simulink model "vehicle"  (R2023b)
settings: Solver=ode3  StartTime=0.0  StopTime=t_end  FixedStep=dt8dof  RelTol=1e-3
PreLoadFcn:
  | define_swarm_buses(3, 1000);
model workspace (MAT data in the model file):
  Af = 1.8
  Cp_tyre = 500
  Cx = 0.28
  G = 15000
  Ha = 0.4
  Hg = 0.4
  Hroll = 0.304
  Hroll_f = 0.08
  Hroll_r = 0.12
  Ir = 0.8
  Ix = 450
  Jz = 1800
  K = 130000
  K_psi = 0.48
  K_y = 0.06
  Karb_F = 26000
  Karb_R = 26000
  KdF = 0
  KdR = 0
  Kd_h = 0
  Kd_v = 0
  Kd_y = 0
  Ki_h = 0
  Ki_v = 0.1
  Ki_y = 0
  Kp_h = 1.5
  Kp_v = 1.5
  Kp_y = 0.1
  Ks_f = 39000
  Ks_r = 39000
  Kv = 290000
  L = 1.5
  Lril_L = 0.055
  Lril_T = 0.5
  MAX_PATH_LEN = 1000
  Pacn = [3000 1 1 1 1 1 1 1 1 0 0 0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]
  R0 = 0.2
  Rfront = 0.2
  Rr_sterzo = 0
  Rrear = 0.2
  Rs = 13
  Tf = 1.5
  Tr = 1.5
  a = 0.6
  a_brake = -3
  b = 0.9
  camb_0F = 0
  camb_0R = -0.00680678408278
  d_max = 0.558505360638
  dt8dof = 0.002
  dtastar = 0.1
  dtcontrol = 0.03
  f0 = 0.0041
  f2 = 2.051e-07
  g = 9.81
  m = 1300
  mot_T_table = [0 0 0 0 0 0 0 0 0 0 0 0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]
  mot_alpha_bp = [0 10 20 30 40 50 60 70 80 90 100]
  mot_n_bp = [0 29.9163426864 59.8326853729 89.7490280593 119.665370746 149.581713432 179.498056119 209.414398805 239.330741492 269.247084178 299.163426864 329.079769551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]
  mpc_speed : object (value not decoded)
  phi_road0 = 0
  psi0 = 0
  r_goal = 5
  r_slow = 30
  replan_steps = 20
  rho = 1.3
  slope_x_body0 = 0
  slope_y_body0 = 0
  t_end = 70
  terrain_truth_mu_table = [-1 -1 -1 -1 -1 -1 -1 -1 -1 -1 -1 -1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]
  terrain_truth_obstacle_table = [1 1 1 1 1 1 1 1 1 1 1 1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]
  terrain_truth_slope_deg_table = [2.67415653197 2.67413215857 2.67406695826 2.6739952249 2.6739164067 2.67382991742 2.67373513563 2.67363140411 2.67351802953 2.67339428225 2.67325939642 2.67311257041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]
  terrain_truth_slope_x_table = [-0.0458815772305 -0.0458808922252 -0.0458794511544 -0.0458778616187 -0.0458761104845 -0.0458741837099 -0.0458720663111 -0.0458697423295 -0.0458671948025 -0.0458644057365 -0.0458613560839 -0.045858025724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]
  terrain_truth_slope_y_table = [0.00874081815183 0.00874213563744 0.00874360556 0.00874524373283 0.00874706738108 0.00874909524079 0.00875134766185 0.00875384671474 0.00875661630067 0.00875968226488 0.00876307251276 0.0087668171283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]
  terrain_truth_traversable_table = [0 0 0 0 0 0 0 0 0 0 0 0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]
  terrain_truth_x_bp = [0 1 2 3 4 5 6 7 8 9 10 11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]
  terrain_truth_y_bp = [0 1 2 3 4 5 6 7 8 9 10 11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]
  teta0 = 0
  tetapunto0 = 0
  theta_road0 = 0
  toe_F = -0.00174532925199
  toe_R = 0.00174532925199
  velstart = 5
  wr0_FL = 3.15
  wr0_FR = 3.15
  wr0_RL = 3.15
  wr0_RR = 3.15
  x0 = 0
  y0 = 0
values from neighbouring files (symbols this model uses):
  gear_ratio = 10    [motor_map.m]
  v_ref_init = scenario.vehicle8.velstart    [make_vref_filter.m]
undefined symbols (not defined in the file or in its folder): A_f, B_f, C_f, D_f, psi0_1
libraries: simulink_extras x15, mpclib x1, slpidlib x1
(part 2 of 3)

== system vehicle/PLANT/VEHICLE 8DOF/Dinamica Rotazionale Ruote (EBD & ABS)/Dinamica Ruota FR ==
  Cm : Inport
  Cf : Inport  Port=2
  Fx : Inport  Port=3
  R : Inport  Port=4
  Fz : Inport  Port=5
  Rr : Inport  Port=6
  Add : Sum  Inputs=+---
  Constant : Constant  Value=velstart
  Divide : Product  Inputs=*/
  FR : Scope
  Integrator2 : Integrator  InitialConditionSource=external  LowerSaturationLimit=0
  Manual Switch : ManualSwitch  CurrentSetting=0
  Mom Inerzia Ruota : Constant  Value=Ir
  Mux : Mux  Inputs=5
  Mux2 : Mux  Inputs=2
  Product3 : Product  RndMeth=Zero
  Product5 : Product  Inputs=*/  RndMeth=Zero
  Resistenza a Rotolmento : Fcn  Expr=u(1)*(f0+f2*u(2)^2)
  Saturation : Saturate  UpperLimit=inf  LowerLimit=0
  cond iniziale wr0 : Constant  Value=wr0_FR
  w : Outport  VectorParamsAs1DForOutWhenUnconnected=off
  R_roll : Outport  Port=2
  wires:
  Resistenza a Rotolmento/1 -> R_roll/1, Add/4, Mux/5
  Mux2/1 -> Resistenza a Rotolmento/1
  Integrator2/1 -> Mux2/2, Saturation/1
  Fz/1 -> Mux2/1
  Product5/1 -> Integrator2/1
  Mom Inerzia Ruota/1 -> Product5/2
  Add/1 -> Product5/1
  Product3/1 -> Add/3, Mux/3
  R/1 -> Product3/2, Mux/4
  Fx/1 -> Product3/1
  Cf/1 -> Add/2, Mux/2
  Cm/1 -> Add/1, Mux/1
  Mux/1 -> FR/1
  Manual Switch/1 -> Integrator2/2
  cond iniziale wr0/1 -> Manual Switch/1
  Saturation/1 -> w/1
  Divide/1 -> Manual Switch/2
  Rr/1 -> Divide/2
  Constant/1 -> Divide/1

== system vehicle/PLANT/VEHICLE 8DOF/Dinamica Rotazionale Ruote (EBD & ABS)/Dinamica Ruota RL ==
  Cm : Inport
  Cf : Inport  Port=2
  Fx : Inport  Port=3
  R : Inport  Port=4
  Fz : Inport  Port=5
  Rr : Inport  Port=6
  Add : Sum  Inputs=+---
  Constant : Constant  Value=velstart
  Divide : Product  Inputs=*/
  Integrator2 : Integrator  InitialConditionSource=external  LowerSaturationLimit=0
  Manual Switch : ManualSwitch  CurrentSetting=0
  Mom Inerzia Ruota : Constant  Value=Ir
  Mux : Mux  Inputs=5
  Mux2 : Mux  Inputs=2
  Product3 : Product  RndMeth=Zero
  Product5 : Product  Inputs=*/  RndMeth=Zero
  RL : Scope
  Resistenza a Rotolmento : Fcn  Expr=u(1)*(f0+f2*u(2)^2)
  Saturation : Saturate  UpperLimit=inf  LowerLimit=0
  cond iniziale wr0 : Constant  Value=wr0_RL
  w : Outport  VectorParamsAs1DForOutWhenUnconnected=off
  R_roll : Outport  Port=2
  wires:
  Resistenza a Rotolmento/1 -> R_roll/1, Add/4, Mux/5
  Mux2/1 -> Resistenza a Rotolmento/1
  Integrator2/1 -> Mux2/2, Saturation/1
  Fz/1 -> Mux2/1
  Product5/1 -> Integrator2/1
  Mom Inerzia Ruota/1 -> Product5/2
  Add/1 -> Product5/1
  Product3/1 -> Add/3
  R/1 -> Product3/2, Mux/4
  Fx/1 -> Mux/3, Product3/1
  Cf/1 -> Add/2, Mux/2
  Cm/1 -> Add/1, Mux/1
  Mux/1 -> RL/1
  Manual Switch/1 -> Integrator2/2
  cond iniziale wr0/1 -> Manual Switch/1
  Saturation/1 -> w/1
  Divide/1 -> Manual Switch/2
  Rr/1 -> Divide/2
  Constant/1 -> Divide/1

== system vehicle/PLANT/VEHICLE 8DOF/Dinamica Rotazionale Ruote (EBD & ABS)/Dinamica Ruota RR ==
  Cm : Inport
  Cf : Inport  Port=2
  Fx : Inport  Port=3
  R : Inport  Port=4
  Fz : Inport  Port=5
  Rr : Inport  Port=6
  Add : Sum  Inputs=+---
  Constant : Constant  Value=velstart
  Divide : Product  Inputs=*/
  Integrator2 : Integrator  InitialConditionSource=external  LowerSaturationLimit=0
  Manual Switch : ManualSwitch  CurrentSetting=0
  Mom Inerzia Ruota : Constant  Value=Ir
  Mux : Mux  Inputs=5
  Mux2 : Mux  Inputs=2
  Product3 : Product  RndMeth=Zero
  Product5 : Product  Inputs=*/  RndMeth=Zero
  RR : Scope
  Resistenza a Rotolmento : Fcn  Expr=u(1)*(f0+f2*u(2)^2)
  Saturation : Saturate  UpperLimit=inf  LowerLimit=0
  cond iniziale wr0 : Constant  Value=wr0_RR
  w : Outport  VectorParamsAs1DForOutWhenUnconnected=off
  R_roll : Outport  Port=2
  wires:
  Resistenza a Rotolmento/1 -> R_roll/1, Add/4, Mux/5
  Mux2/1 -> Resistenza a Rotolmento/1
  Integrator2/1 -> Mux2/2, Saturation/1
  Fz/1 -> Mux2/1
  Product5/1 -> Integrator2/1
  Mom Inerzia Ruota/1 -> Product5/2
  Add/1 -> Product5/1
  Product3/1 -> Add/3
  R/1 -> Product3/2, Mux/4
  Fx/1 -> Mux/3, Product3/1
  Cf/1 -> Add/2, Mux/2
  Cm/1 -> Add/1, Mux/1
  Mux/1 -> RR/1
  Manual Switch/1 -> Integrator2/2
  cond iniziale wr0/1 -> Manual Switch/1
  Saturation/1 -> w/1
  Divide/1 -> Manual Switch/2
  Rr/1 -> Divide/2
  Constant/1 -> Divide/1

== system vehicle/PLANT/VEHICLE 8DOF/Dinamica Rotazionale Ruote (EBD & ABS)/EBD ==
  %brake : Inport
  mu : Inport  Port=2
  Fz : Inport  Port=3
  Add : Sum  Inputs=++++
  Demux : Demux
  Divide{,1..3} (4 alike) : Product  Inputs=*/
  Gain : Gain  Gain=1.5
  Mux : Mux
  Product{,1..4} (5 alike) : Product
  Saturation : Saturate  UpperLimit=inf  LowerLimit=.05
  Saturation1 : Saturate  UpperLimit=inf  LowerLimit=50
  Saturation2 : Saturate  UpperLimit=inf  LowerLimit=eps
  Cf : Outport
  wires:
  mu/1 -> Saturation/1
  Fz/1 -> Saturation1/1
  Product/1 -> Demux/1
  Demux/1 -> Divide/1, Add/1
  Saturation/1 -> Product/1
  Saturation1/1 -> Product/2
  Demux/2 -> Divide1/1, Add/2
  Demux/3 -> Divide2/1, Add/3
  Demux/4 -> Divide3/1, Add/4
  Add/1 -> Saturation2/1
  Saturation2/1 -> Divide3/2, Divide2/2, Divide1/2, Divide/2
  Divide/1 -> Product1/1
  %brake/1 -> Product4/2, Product3/2, Product2/2, Product1/2
  Divide1/1 -> Product2/1
  Divide2/1 -> Product3/1
  Divide3/1 -> Product4/1
  Product1/1 -> Mux/1
  Product2/1 -> Mux/2
  Product3/1 -> Mux/3
  Product4/1 -> Mux/4
  Mux/1 -> Gain/1
  Gain/1 -> Cf/1

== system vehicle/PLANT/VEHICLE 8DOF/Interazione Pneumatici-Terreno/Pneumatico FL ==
  vel_x : Inport
  R : Inport  Port=2
  alfa : Inport  Port=3
  Fz : Inport  Port=4
  mu_strada : Inport  Port=5
  w : Inport  Port=6
  Calcolo FORZA LATERALE & LONGITUDINALE (Pneumatico - Terreno) : Subsystem
  Gain : Gain  Gain=-1
  Lunghezze di rilassamento : Subsystem
  Radians to Degrees : simulink_extras/Transformations/Radians to Degrees
  Scorrimento : Subsystem
  Fx_rit : Outport  VectorParamsAs1DForOutWhenUnconnected=off
  Fy_rit : Outport  Port=2  VectorParamsAs1DForOutWhenUnconnected=off
  slip_FL : Outport  Port=3
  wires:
  vel_x/1 -> Scorrimento/1(vel_x_cr), Lunghezze di rilassamento/1(vel_x_CR), Calcolo FORZA LATERALE & LONGITUDINALE (Pneumatico - Terreno)/1(Vcx)
  R/1 -> Scorrimento/2(R)
  w/1 -> Scorrimento/3(w)
  Calcolo FORZA LATERALE & LONGITUDINALE (Pneumatico - Terreno)/1(Fy) -> Lunghezze di rilassamento/2(Fy)
  Calcolo FORZA LATERALE & LONGITUDINALE (Pneumatico - Terreno)/2(Fx) -> Lunghezze di rilassamento/3(Fx)
  Scorrimento/1(s) -> slip_FL/1, Calcolo FORZA LATERALE & LONGITUDINALE (Pneumatico - Terreno)/3(s)
  alfa/1 -> Radians to Degrees/1
  Fz/1 -> Calcolo FORZA LATERALE & LONGITUDINALE (Pneumatico - Terreno)/4(Fz)
  Lunghezze di rilassamento/1(Fy_rit) -> Gain/1
  mu_strada/1 -> Calcolo FORZA LATERALE & LONGITUDINALE (Pneumatico - Terreno)/2(mu_strada)
  Radians to Degrees/1 -> Calcolo FORZA LATERALE & LONGITUDINALE (Pneumatico - Terreno)/5(alfa)
  Gain/1 -> Fy_rit/1
  Lunghezze di rilassamento/2(Fx_rit) -> Fx_rit/1

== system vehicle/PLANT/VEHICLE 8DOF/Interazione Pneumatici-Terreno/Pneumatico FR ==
  vel_x : Inport
  R : Inport  Port=2
  alfa : Inport  Port=3
  Fz : Inport  Port=4
  mu_strada : Inport  Port=5
  w : Inport  Port=6
  Calcolo FORZA LATERALE & LONGITUDINALE (Pneumatico - Terreno) : Subsystem
  First Order Hold1 : FirstOrderHold  Commented=through  ErrorTolerance=inf  AllowContinuousInput=on
  First Order Hold2 : FirstOrderHold  Commented=through  ErrorTolerance=inf  AllowContinuousInput=on
  Gain : Gain  Gain=-1
  Lunghezze di rilassamento : Subsystem
  Radians to Degrees : simulink_extras/Transformations/Radians to Degrees
  Scorrimento : Subsystem
  Fx_rit : Outport  VectorParamsAs1DForOutWhenUnconnected=off
  Fy_rit : Outport  Port=2  VectorParamsAs1DForOutWhenUnconnected=off
  slip_FR : Outport  Port=3
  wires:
  vel_x/1 -> Scorrimento/1(vel_x_cr), Calcolo FORZA LATERALE & LONGITUDINALE (Pneumatico - Terreno)/1(Vcx), Lunghezze di rilassamento/1(vel_x_CR)
  R/1 -> Scorrimento/2(R)
  w/1 -> Scorrimento/3(w)
  Calcolo FORZA LATERALE & LONGITUDINALE (Pneumatico - Terreno)/1(Fy) -> Lunghezze di rilassamento/2(Fy)
  Calcolo FORZA LATERALE & LONGITUDINALE (Pneumatico - Terreno)/2(Fx) -> Lunghezze di rilassamento/3(Fx)
  Scorrimento/1(s) -> slip_FR/1, Calcolo FORZA LATERALE & LONGITUDINALE (Pneumatico - Terreno)/3(s)
  alfa/1 -> Radians to Degrees/1
  Fz/1 -> Calcolo FORZA LATERALE & LONGITUDINALE (Pneumatico - Terreno)/4(Fz)
  Lunghezze di rilassamento/1(Fy_rit) -> Gain/1
  Lunghezze di rilassamento/2(Fx_rit) -> First Order Hold2/1
  mu_strada/1 -> Calcolo FORZA LATERALE & LONGITUDINALE (Pneumatico - Terreno)/2(mu_strada)
  Radians to Degrees/1 -> Calcolo FORZA LATERALE & LONGITUDINALE (Pneumatico - Terreno)/5(alfa)
  Gain/1 -> First Order Hold1/1
  First Order Hold1/1 -> Fy_rit/1
  First Order Hold2/1 -> Fx_rit/1

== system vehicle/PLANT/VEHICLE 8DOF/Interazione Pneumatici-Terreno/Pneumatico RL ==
  vel_x : Inport
  R : Inport  Port=2
  alfa : Inport  Port=3
  Fz : Inport  Port=4
  mu_strada : Inport  Port=5
  w : Inport  Port=6
  Calcolo FORZA LATERALE & LONGITUDINALE (Pneumatico - Terreno) : Subsystem
  First Order Hold1 : FirstOrderHold  Commented=through  ErrorTolerance=inf  AllowContinuousInput=on
  First Order Hold2 : FirstOrderHold  Commented=through  ErrorTolerance=inf  AllowContinuousInput=on
  Gain : Gain  Gain=-1
  Lunghezze di rilassamento : Subsystem
  Radians to Degrees : simulink_extras/Transformations/Radians to Degrees
  Scorrimento : Subsystem
  Fx_rit : Outport  VectorParamsAs1DForOutWhenUnconnected=off
  Fy_rit : Outport  Port=2  VectorParamsAs1DForOutWhenUnconnected=off
  slip_RL : Outport  Port=3
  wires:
  vel_x/1 -> Scorrimento/1(vel_x_cr), Calcolo FORZA LATERALE & LONGITUDINALE (Pneumatico - Terreno)/1(Vcx), Lunghezze di rilassamento/1(vel_x_CR)
  R/1 -> Scorrimento/2(R)
  w/1 -> Scorrimento/3(w)
  Calcolo FORZA LATERALE & LONGITUDINALE (Pneumatico - Terreno)/1(Fy) -> Lunghezze di rilassamento/2(Fy)
  Calcolo FORZA LATERALE & LONGITUDINALE (Pneumatico - Terreno)/2(Fx) -> Lunghezze di rilassamento/3(Fx)
  Scorrimento/1(s) -> slip_RL/1, Calcolo FORZA LATERALE & LONGITUDINALE (Pneumatico - Terreno)/3(s)
  alfa/1 -> Radians to Degrees/1
  Fz/1 -> Calcolo FORZA LATERALE & LONGITUDINALE (Pneumatico - Terreno)/4(Fz)
  Lunghezze di rilassamento/1(Fy_rit) -> Gain/1
  Lunghezze di rilassamento/2(Fx_rit) -> First Order Hold2/1
  mu_strada/1 -> Calcolo FORZA LATERALE & LONGITUDINALE (Pneumatico - Terreno)/2(mu_strada)
  Radians to Degrees/1 -> Calcolo FORZA LATERALE & LONGITUDINALE (Pneumatico - Terreno)/5(alfa)
  Gain/1 -> First Order Hold1/1
  First Order Hold1/1 -> Fy_rit/1
  First Order Hold2/1 -> Fx_rit/1

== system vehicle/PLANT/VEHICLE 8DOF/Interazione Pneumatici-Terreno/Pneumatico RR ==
  vel_x : Inport
  R : Inport  Port=2
  alfa : Inport  Port=3
  Fz : Inport  Port=4
  mu_strada : Inport  Port=5
  w : Inport  Port=6
  Calcolo FORZA LATERALE & LONGITUDINALE (Pneumatico - Terreno) : Subsystem
  First Order Hold1 : FirstOrderHold  Commented=through  ErrorTolerance=inf  AllowContinuousInput=on
  First Order Hold2 : FirstOrderHold  Commented=through  ErrorTolerance=inf  AllowContinuousInput=on
  Gain : Gain  Gain=-1
  Lunghezze di rilassamento : Subsystem
  Radians to Degrees : simulink_extras/Transformations/Radians to Degrees
  Scorrimento : Subsystem
  Fx_rit : Outport  VectorParamsAs1DForOutWhenUnconnected=off
  Fy_rit : Outport  Port=2  VectorParamsAs1DForOutWhenUnconnected=off
  slip_RR : Outport  Port=3
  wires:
  vel_x/1 -> Scorrimento/1(vel_x_cr), Calcolo FORZA LATERALE & LONGITUDINALE (Pneumatico - Terreno)/1(Vcx), Lunghezze di rilassamento/1(vel_x_CR)
  R/1 -> Scorrimento/2(R)
  w/1 -> Scorrimento/3(w)
  Calcolo FORZA LATERALE & LONGITUDINALE (Pneumatico - Terreno)/1(Fy) -> Lunghezze di rilassamento/2(Fy)
  Calcolo FORZA LATERALE & LONGITUDINALE (Pneumatico - Terreno)/2(Fx) -> Lunghezze di rilassamento/3(Fx)
  Scorrimento/1(s) -> slip_RR/1, Calcolo FORZA LATERALE & LONGITUDINALE (Pneumatico - Terreno)/3(s)
  alfa/1 -> Radians to Degrees/1
  Fz/1 -> Calcolo FORZA LATERALE & LONGITUDINALE (Pneumatico - Terreno)/4(Fz)
  Lunghezze di rilassamento/1(Fy_rit) -> Gain/1
  Lunghezze di rilassamento/2(Fx_rit) -> First Order Hold2/1
  mu_strada/1 -> Calcolo FORZA LATERALE & LONGITUDINALE (Pneumatico - Terreno)/2(mu_strada)
  Radians to Degrees/1 -> Calcolo FORZA LATERALE & LONGITUDINALE (Pneumatico - Terreno)/5(alfa)
  Gain/1 -> First Order Hold1/1
  First Order Hold1/1 -> Fy_rit/1
  First Order Hold2/1 -> Fx_rit/1

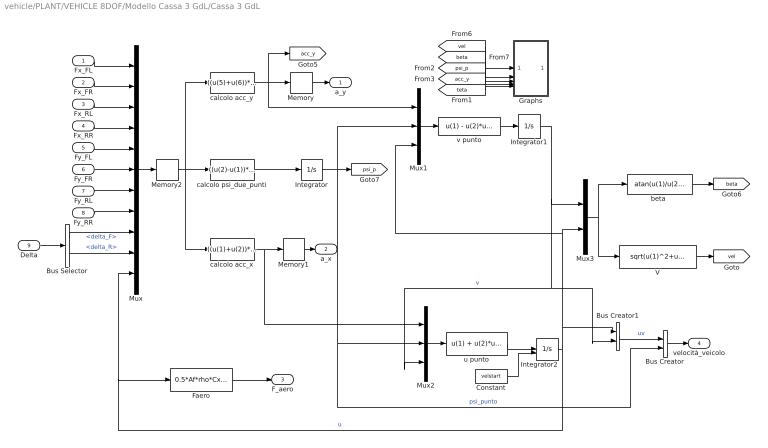
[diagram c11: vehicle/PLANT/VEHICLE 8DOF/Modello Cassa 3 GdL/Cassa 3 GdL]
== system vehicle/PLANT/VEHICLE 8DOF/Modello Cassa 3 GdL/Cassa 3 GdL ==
  Fx_FL : Inport
  Fx_FR : Inport  Port=2
  Fx_RL : Inport  Port=3
  Fx_RR : Inport  Port=4
  Fy_FL : Inport  Port=5
  Fy_FR : Inport  Port=6
  Fy_RL : Inport  Port=7
  Fy_RR : Inport  Port=8
  Delta : Inport  Port=9
  Bus Creator : BusCreator  Inputs=2
  Bus Creator1 : BusCreator  Inputs=2
  Bus Selector : BusSelector  OutputSignals=delta_F,delta_R
  Constant : Constant  Value=velstart
  Faero : Fcn  Expr=0.5*Af*rho*Cx*u^2
  Graphs : Subsystem  Commented=on
  Integrator : Integrator
  Integrator1 : Integrator
  Integrator2 : Integrator  InitialConditionSource=external  InitialCondition=velstart  LimitOutput=on  LowerSaturationLimit=eps
  Memory : Memory  Commented=through
  Memory1 : Memory  Commented=through
  Memory2 : Memory  Commented=through
  Mux : Mux  Inputs=11
  Mux1 : Mux  Inputs=3
  Mux2 : Mux  Inputs=3
  Mux3 : Mux  Inputs=2
  V : Fcn  Expr=sqrt(u(1)^2+u(2)^2)
  "beta " : Fcn  Expr=atan(u(1)/u(2))
  calcolo acc_x : Fcn  Expr=((u(1)+u(2))*cos(u(9))+(u(3)+u(4))*cos(u(10))-(u(5)+u(6))*sin(u(9))-(u(7)+u(8))*sin(u(10))-(0.5*Af*rho*Cx*(u(11)^2)))/m
  calcolo acc_y : Fcn  Expr=((u(5)+u(6))*cos(u(9))+(u(7)+u(8))*cos(u(10))+(u(1)+u(2))*sin(u(9))+(u(3)+u(4))*sin(u(10)))/m
  calcolo psi_due_punti : Fcn  Expr=((u(2)-u(1))*(Tf/2)*cos(u(9))+(u(4)-u(3))*(Tr/2)*cos(u(10))+(u(1)+u(2))*a*sin(u(9))-(u(3)+u(4))*b*sin(u(10))+(u(6)+u(5))*a*cos(u(9))-(u(7)+u(8))*b*cos(u(10))-(u(6)-u(5))*(Tf/2)*sin(u(9))+(u(7)-u(8))*(Tr/2)*sin(u(10)))/Jz
  u punto : Fcn  Expr=u(1) + u(2)*u(3)
  v punto : Fcn  Expr=u(1) - u(2)*u(3)
  a_y : Outport  VectorParamsAs1DForOutWhenUnconnected=off
  a_x : Outport  Port=2  VectorParamsAs1DForOutWhenUnconnected=off
  F_aero : Outport  Port=3  VectorParamsAs1DForOutWhenUnconnected=off
  velocità_veicolo : Outport  Port=4
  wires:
  Fx_FL/1 -> Mux/1
  Fx_FR/1 -> Mux/2
  Fx_RL/1 -> Mux/3
  Fx_RR/1 -> Mux/4
  Fy_FL/1 -> Mux/5
  Fy_FR/1 -> Mux/6
  Fy_RL/1 -> Mux/7
  Fy_RR/1 -> Mux/8
  Bus Selector/2 -> Mux/10  "<delta_R>"
  Mux/1 -> Memory2/1
  calcolo acc_y/1 -> [acc_y], Mux1/1, Memory/1
  calcolo psi_due_punti/1 -> Integrator/1
  calcolo acc_x/1 -> Mux2/1, Memory1/1
  Mux2/1 -> u punto/1
  Mux1/1 -> v punto/1
  u punto/1 -> Integrator2/1
  v punto/1 -> Integrator1/1
  Mux3/1 -> "beta "/1, V/1
  V/1 -> [vel]
  Memory/1 -> a_y/1
  Memory1/1 -> a_x/1
  Faero/1 -> F_aero/1
  Bus Creator/1 -> velocità_veicolo/1
  Bus Creator1/1 -> Bus Creator/1  "uv"
  Integrator1/1 -> Mux3/1, Bus Creator1/2, Mux2/3  "v"
  Integrator2/1 -> Bus Creator1/1, Mux1/3, Mux3/2, Mux/11, Faero/1  "u"
  Integrator/1 -> [psi_p], Mux2/2, Bus Creator/2, Mux1/2  "psi_punto"
  [psi_p] -> Graphs/3(psi_p)
  [vel] -> Graphs/1(vel)
  [beta] -> Graphs/2(beta)
  [teta] -> Graphs/5(teta)
  [acc_y] -> Graphs/4(a_y)
  "beta "/1 -> [beta]
  Delta/1 -> Bus Selector/1
  Bus Selector/1 -> Mux/9  "<delta_F>"
  Constant/1 -> Integrator2/2
  Memory2/1 -> calcolo psi_due_punti/1, calcolo acc_y/1, calcolo acc_x/1

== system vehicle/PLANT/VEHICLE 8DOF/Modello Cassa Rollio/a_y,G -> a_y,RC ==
  teta_pp : Inport
  a_y,G : Inport  Port=2
  "teta " : Inport  Port=3
  Add2 : Sum
  "Distanza CG-CR " : Constant  Value=Hroll
  Divide : Product  Inputs=***
  Trigonometric Function2 : Trigonometry  Operator=cos
  a_y,RC : Outport  VectorParamsAs1DForOutWhenUnconnected=off
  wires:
  Trigonometric Function2/1 -> Divide/3
  "Distanza CG-CR "/1 -> Divide/2
  teta_pp/1 -> Divide/1
  "teta "/1 -> Trigonometric Function2/1
  a_y,G/1 -> Add2/1
  Divide/1 -> Add2/2
  Add2/1 -> a_y,RC/1

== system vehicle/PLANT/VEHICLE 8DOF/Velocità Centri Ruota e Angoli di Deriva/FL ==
  delta : Inport
  u_cr : Inport  Port=2
  v_cr : Inport  Port=3
  Add : Sum  Inputs=-+
  Mux2 : Mux  Inputs=2
  Product : Product  RndMeth=Zero
  Scope{,1..4} (5 alike) : Scope
  Trigonometric Function : Trigonometry  Operator=cos
  "V_cr " : Fcn  Expr=sqrt(u(1)^2+u(2)^2)
  num atan1 : Fcn  Expr=atan (u(2)/u(1))
  alfa : Outport  VectorParamsAs1DForOutWhenUnconnected=off
  vel_x_cr : Outport  Port=2  VectorParamsAs1DForOutWhenUnconnected=off
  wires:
  v_cr/1 -> Scope3/1, Mux2/2
  u_cr/1 -> Scope2/1, Mux2/1
  Mux2/1 -> num atan1/1, "V_cr "/1
  num atan1/1 -> Scope4/1, Add/2  "gamma"
  Add/1 -> alfa/1, Trigonometric Function/1, Scope1/1
  Trigonometric Function/1 -> Product/1
  "V_cr "/1 -> Product/2  "V_cr"
  Product/1 -> vel_x_cr/1
  delta/1 -> Scope/1, Add/1

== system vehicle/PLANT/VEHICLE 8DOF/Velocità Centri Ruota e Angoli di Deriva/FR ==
  delta : Inport
  u_cr : Inport  Port=2
  v_cr : Inport  Port=3
  Add : Sum  Inputs=-+
  Mux2 : Mux  Inputs=2
  Product : Product  RndMeth=Zero
  Trigonometric Function : Trigonometry  Operator=cos
  "V_cr " : Fcn  Expr=sqrt(u(1)^2+u(2)^2)
  num atan1 : Fcn  Expr=atan (u(2)/u(1))
  alfa : Outport  VectorParamsAs1DForOutWhenUnconnected=off
  vel_x_cr : Outport  Port=2  VectorParamsAs1DForOutWhenUnconnected=off
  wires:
  v_cr/1 -> Mux2/2
  u_cr/1 -> Mux2/1
  delta/1 -> Add/1
  Mux2/1 -> num atan1/1, "V_cr "/1
  num atan1/1 -> Add/2  "gamma"
  Add/1 -> Trigonometric Function/1, alfa/1
  Trigonometric Function/1 -> Product/1
  "V_cr "/1 -> Product/2  "V_cr"
  Product/1 -> vel_x_cr/1

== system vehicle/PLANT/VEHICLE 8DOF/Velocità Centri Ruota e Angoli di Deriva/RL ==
  delta : Inport
  u_cr : Inport  Port=2
  v_cr : Inport  Port=3
  Add : Sum  Inputs=-+
  Mux2 : Mux  Inputs=2
  Product : Product  RndMeth=Zero
  Trigonometric Function : Trigonometry  Operator=cos
  "V_cr " : Fcn  Expr=sqrt(u(1)^2+u(2)^2)
  num atan1 : Fcn  Expr=atan (u(2)/u(1))
  alfa : Outport  VectorParamsAs1DForOutWhenUnconnected=off
  vel_x_cr : Outport  Port=2  VectorParamsAs1DForOutWhenUnconnected=off
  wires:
  v_cr/1 -> Mux2/2
  u_cr/1 -> Mux2/1
  delta/1 -> Add/1
  Mux2/1 -> num atan1/1, "V_cr "/1
  num atan1/1 -> Add/2  "gamma"
  Add/1 -> Trigonometric Function/1, alfa/1
  Trigonometric Function/1 -> Product/1
  "V_cr "/1 -> Product/2  "V_cr"
  Product/1 -> vel_x_cr/1

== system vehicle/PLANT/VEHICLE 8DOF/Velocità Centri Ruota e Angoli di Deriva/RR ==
  delta : Inport
  u_cr : Inport  Port=2
  v_cr : Inport  Port=3
  Add : Sum  Inputs=-+
  Mux2 : Mux  Inputs=2
  Product : Product  RndMeth=Zero
  Trigonometric Function : Trigonometry  Operator=cos
  "V_cr " : Fcn  Expr=sqrt(u(1)^2+u(2)^2)
  num atan1 : Fcn  Expr=atan (u(2)/u(1))
  alfa : Outport  VectorParamsAs1DForOutWhenUnconnected=off
  vel_x_cr : Outport  Port=2  VectorParamsAs1DForOutWhenUnconnected=off
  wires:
  v_cr/1 -> Mux2/2
  u_cr/1 -> Mux2/1
  delta/1 -> Add/1
  Mux2/1 -> num atan1/1, "V_cr "/1
  num atan1/1 -> Add/2  "gamma"
  Add/1 -> Trigonometric Function/1, alfa/1
  Trigonometric Function/1 -> Product/1
  "V_cr "/1 -> Product/2  "V_cr"
  Product/1 -> vel_x_cr/1

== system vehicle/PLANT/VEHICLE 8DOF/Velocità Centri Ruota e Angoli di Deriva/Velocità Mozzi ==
  velocità_veicolo : Inport
  Bus Selector : BusSelector  OutputSignals=uv.u,uv.v,psi_punto
  Mux5 : Mux  Inputs=3
  u_cr : Fcn  Expr=u(1) - u(3)*Tf/2
  u_cr1 : Fcn  Expr=u(1) - u(3)*Tr/2
  u_cr2 : Fcn  Expr=u(1) + u(3)*Tf/2
  u_cr3 : Fcn  Expr=u(1) + u(3)*Tr/2
  v_cr : Fcn  Expr=u(2) + u(3)*a
  v_cr1 : Fcn  Expr=u(2) - u(3)*b
  v_cr2 : Fcn  Expr=u(2) + u(3)*a
  v_cr3 : Fcn  Expr=u(2) - u(3)*b
  "u_FL " : Outport  VectorParamsAs1DForOutWhenUnconnected=off
  "v_FL " : Outport  Port=2  VectorParamsAs1DForOutWhenUnconnected=off
  u_FR : Outport  Port=3  VectorParamsAs1DForOutWhenUnconnected=off
  v_FR : Outport  Port=4  VectorParamsAs1DForOutWhenUnconnected=off
  u _RL : Outport  Port=5  VectorParamsAs1DForOutWhenUnconnected=off
  v_RL : Outport  Port=6  VectorParamsAs1DForOutWhenUnconnected=off
  u_RR : Outport  Port=7  VectorParamsAs1DForOutWhenUnconnected=off
  v_RR : Outport  Port=8  VectorParamsAs1DForOutWhenUnconnected=off
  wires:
  Bus Selector/3 -> Mux5/3  "<psi_punto>"
  Bus Selector/2 -> Mux5/2  "<v>"
  Bus Selector/1 -> Mux5/1  "<u>"
  Mux5/1 -> v_cr/1, u_cr/1, u_cr3/1, v_cr3/1, v_cr2/1, u_cr2/1, u_cr1/1, v_cr1/1
  u_cr3/1 -> u_RR/1  "u_RR"
  v_cr3/1 -> v_RR/1  "v_RR"
  v_cr2/1 -> v_FR/1  "v_FR"
  u_cr2/1 -> u_FR/1  "u_FR"
  v_cr1/1 -> v_RL/1  "v_RL"
  u_cr1/1 -> u _RL/1  "u_RL"
  v_cr/1 -> "v_FL "/1  "v_FL"
  u_cr/1 -> "u_FL "/1  "u_FL"
  velocità_veicolo/1 -> Bus Selector/1

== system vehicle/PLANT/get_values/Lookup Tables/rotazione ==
  slope xabs : Inport
  slope yabs : Inport  Port=2
  -psi : Inport  Port=3
  Cos : Trigonometry  Operator=cos
  Minus1 : Sum
  Minus3 : Sum  Inputs=+-
  Product{,1..3} (4 alike) : Product
  Sin : Trigonometry
  slope x vehicle : Outport
  slope y vehicle : Outport  Port=2
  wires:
  Product2/1 -> Minus1/1
  Product3/1 -> Minus1/2
  Cos/1 -> Product3/1, Product/2
  slope yabs/1 -> Product3/2, Product1/1
  Sin/1 -> Product2/2, Product1/2
  slope xabs/1 -> Product/1, Product2/1
  Product1/1 -> Minus3/2
  Product/1 -> Minus3/1
  Minus3/1 -> slope x vehicle/1  "x_dot"
  Minus1/1 -> slope y vehicle/1  "y_dot"
  -psi/1 -> Sin/1, Cos/1

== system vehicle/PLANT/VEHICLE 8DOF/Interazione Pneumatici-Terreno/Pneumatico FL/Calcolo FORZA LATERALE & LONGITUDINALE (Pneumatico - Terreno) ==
  Vcx : Inport
  mu_strada : Inport  Port=2
  s : Inport  Port=3
  Fz : Inport  Port=4
  alfa : Inport  Port=5
  Camber : Constant  Value=0
  Constant : Constant  Value=Pacn
  Degrees to Radians : simulink_extras/Transformations/Degrees to Radians
  Degrees to Radians1 : simulink_extras/Transformations/Degrees to Radians
  Demux : Demux  Outputs=3
  Gain : Gain  Gain=-1
  Pacejka 96 : MATLAB Function  TreatAsAtomicUnit=on
  Terminator : Terminator
  Terminator1 : Terminator
  raggio ruota scarica [m] : Constant  Value=Rfront
  Fy : Outport  VectorParamsAs1DForOutWhenUnconnected=off
  Fx : Outport  Port=2  VectorParamsAs1DForOutWhenUnconnected=off
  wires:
  Demux/2 -> Gain/1  "Fy"
  Demux/1 -> Fx/1  "Fx"
  raggio ruota scarica [m]/1 -> Pacejka 96/8(R0)
  Vcx/1 -> Pacejka 96/7(Vcx)
  Degrees to Radians1/1 -> Pacejka 96/4(alfa)
  Degrees to Radians/1 -> Pacejka 96/2(gamma)
  Constant/1 -> Pacejka 96/1(Pac)
  Pacejka 96/1(F_pac) -> Demux/1
  Demux/3 -> Terminator1/1  "Mz"
  Pacejka 96/2(C_F) -> Terminator/1
  Camber/1 -> Degrees to Radians/1
  mu_strada/1 -> Pacejka 96/6(mu)
  s/1 -> Pacejka 96/3(slip)
  Fz/1 -> Pacejka 96/5(Fz)
  alfa/1 -> Degrees to Radians1/1
  Gain/1 -> Fy/1

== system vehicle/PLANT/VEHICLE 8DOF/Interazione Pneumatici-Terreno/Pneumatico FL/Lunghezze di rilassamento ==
  vel_x_CR : Inport
  Fy : Inport  Port=2
  Fx : Inport  Port=3
  Integrator : Integrator
  Integrator1 : Integrator
  Lunghezza di rilassamento longitudinale : Constant  Value=Lril_L
  Lunghezza di rilassamento trasversale : Constant  Value=Lril_T
  Math Function : Math  Operator=reciprocal  SignedPower=on
  Math Function1 : Math  Operator=reciprocal  SignedPower=on
  Product{,1..3} (4 alike) : Product  InputSameDT=on  SaturateOnIntegerOverflow=on
  Sum1 : Sum  Inputs=-+  InputSameDT=on  SaturateOnIntegerOverflow=on
  Sum2 : Sum  Inputs=-+  InputSameDT=on  SaturateOnIntegerOverflow=on
  Fy_rit : Outport  VectorParamsAs1DForOutWhenUnconnected=off
  Fx_rit : Outport  Port=2  VectorParamsAs1DForOutWhenUnconnected=off
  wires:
  Lunghezza di rilassamento longitudinale/1 -> Math Function/1
  Fx/1 -> Sum1/2
  Product/1 -> Product1/2
  Sum1/1 -> Product1/1
  Product1/1 -> Integrator/1
  Integrator/1 -> Fx_rit/1, Sum1/1
  vel_x_CR/1 -> Product/2, Product2/2
  Lunghezza di rilassamento trasversale/1 -> Math Function1/1
  Math Function1/1 -> Product2/1
  Fy/1 -> Sum2/2
  Product2/1 -> Product3/2
  Sum2/1 -> Product3/1
  Product3/1 -> Integrator1/1
  Integrator1/1 -> Fy_rit/1, Sum2/1
  Math Function/1 -> Product/1

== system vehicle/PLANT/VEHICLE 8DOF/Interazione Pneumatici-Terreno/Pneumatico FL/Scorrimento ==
  vel_x_cr : Inport
  R : Inport  Port=2
  w : Inport  Port=3
  Mux9 : Mux  Inputs=2
  Product : Product  InputSameDT=on  SaturateOnIntegerOverflow=on
  Switch : Switch
  slip frenata : Fcn  Expr=(u[2]/(u[1]+(u[1]==0)*eps))-1
  "slip trazione (GIUSTO, LA FUNZIONE NON SERVE)" : Fcn  Expr=1-(u[1]/(u[2]+(u[2]==0)*eps))
  s : Outport  VectorParamsAs1DForOutWhenUnconnected=off
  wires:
  slip frenata/1 -> Switch/3
  Mux9/1 -> slip frenata/1, "slip trazione (GIUSTO, LA FUNZIONE NON SERVE)"/1
  vel_x_cr/1 -> Mux9/1
  Switch/1 -> s/1
  Product/1 -> Mux9/2
  w/1 -> Product/1
  R/1 -> Product/2
  "slip trazione (GIUSTO, LA FUNZIONE NON SERVE)"/1 -> Switch/1, Switch/2

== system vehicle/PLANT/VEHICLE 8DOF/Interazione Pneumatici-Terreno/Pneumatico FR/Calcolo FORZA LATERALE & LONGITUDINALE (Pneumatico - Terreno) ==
  Vcx : Inport
  mu_strada : Inport  Port=2
  s : Inport  Port=3
  Fz : Inport  Port=4
  alfa : Inport  Port=5
  Camber : Constant  Value=0
  Constant : Constant  Value=Pacn
  Degrees to Radians : simulink_extras/Transformations/Degrees to Radians
  Degrees to Radians1 : simulink_extras/Transformations/Degrees to Radians
  Demux : Demux  Outputs=3
  Gain : Gain  Gain=-1
  Pacejka 96 : MATLAB Function  TreatAsAtomicUnit=on
  Terminator : Terminator
  Terminator1 : Terminator
  raggio ruota scarica [m] : Constant  Value=Rfront
  Fy : Outport  VectorParamsAs1DForOutWhenUnconnected=off
  Fx : Outport  Port=2  VectorParamsAs1DForOutWhenUnconnected=off
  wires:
  Demux/2 -> Gain/1  "Fy"
  Demux/1 -> Fx/1  "Fx"
  Constant/1 -> Pacejka 96/1(Pac)
  Pacejka 96/1(F_pac) -> Demux/1
  Degrees to Radians/1 -> Pacejka 96/2(gamma)
  raggio ruota scarica [m]/1 -> Pacejka 96/8(R0)
  Vcx/1 -> Pacejka 96/7(Vcx)
  Fz/1 -> Pacejka 96/5(Fz)
  alfa/1 -> Degrees to Radians1/1
  s/1 -> Pacejka 96/3(slip)
  mu_strada/1 -> Pacejka 96/6(mu)
  Camber/1 -> Degrees to Radians/1
  Demux/3 -> Terminator/1  "Mz"
  Pacejka 96/2(C_F) -> Terminator1/1
  Degrees to Radians1/1 -> Pacejka 96/4(alfa)
  Gain/1 -> Fy/1

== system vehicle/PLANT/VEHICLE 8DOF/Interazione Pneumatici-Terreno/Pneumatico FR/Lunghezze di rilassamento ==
  vel_x_CR : Inport
  Fy : Inport  Port=2
  Fx : Inport  Port=3
  Integrator : Integrator
  Integrator1 : Integrator
  Lunghezza di rilassamento longitudinale : Constant  Value=Lril_L
  Lunghezza di rilassamento trasversale : Constant  Value=Lril_T
  Math Function : Math  Operator=reciprocal  SignedPower=on
  Math Function1 : Math  Operator=reciprocal  SignedPower=on
  Product{,1..3} (4 alike) : Product  InputSameDT=on  SaturateOnIntegerOverflow=on
  Sum1 : Sum  Inputs=-+  InputSameDT=on  SaturateOnIntegerOverflow=on
  Sum2 : Sum  Inputs=-+  InputSameDT=on  SaturateOnIntegerOverflow=on
  Fy_rit : Outport  VectorParamsAs1DForOutWhenUnconnected=off
  Fx_rit : Outport  Port=2  VectorParamsAs1DForOutWhenUnconnected=off
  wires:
  Lunghezza di rilassamento longitudinale/1 -> Math Function/1
  Fx/1 -> Sum1/2
  Product/1 -> Product1/2
  Sum1/1 -> Product1/1
  Product1/1 -> Integrator/1
  Integrator/1 -> Fx_rit/1, Sum1/1
  vel_x_CR/1 -> Product/2, Product2/2
  Lunghezza di rilassamento trasversale/1 -> Math Function1/1
  Math Function1/1 -> Product2/1
  Fy/1 -> Sum2/2
  Product2/1 -> Product3/2
  Sum2/1 -> Product3/1
  Product3/1 -> Integrator1/1
  Integrator1/1 -> Fy_rit/1, Sum2/1
  Math Function/1 -> Product/1

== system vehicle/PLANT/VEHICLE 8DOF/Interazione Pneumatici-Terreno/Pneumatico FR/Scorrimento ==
  vel_x_cr : Inport
  R : Inport  Port=2
  w : Inport  Port=3
  Mux9 : Mux  Inputs=2
  Product : Product  InputSameDT=on  SaturateOnIntegerOverflow=on
  Switch : Switch
  slip frenata : Fcn  Expr=(u[2]/(u[1]+(u[1]==0)*eps))-1
  slip trazione : Fcn  Expr=1-(u[1]/(u[2]+(u[2]==0)*eps))
  s : Outport  VectorParamsAs1DForOutWhenUnconnected=off
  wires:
  slip frenata/1 -> Switch/3
  slip trazione/1 -> Switch/2, Switch/1
  Mux9/1 -> slip frenata/1, slip trazione/1
  vel_x_cr/1 -> Mux9/1
  Switch/1 -> s/1
  Product/1 -> Mux9/2
  w/1 -> Product/1
  R/1 -> Product/2

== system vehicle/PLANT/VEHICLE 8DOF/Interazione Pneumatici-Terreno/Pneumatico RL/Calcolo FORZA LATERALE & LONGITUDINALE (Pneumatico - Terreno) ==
  Vcx : Inport
  mu_strada : Inport  Port=2
  s : Inport  Port=3
  Fz : Inport  Port=4
  alfa : Inport  Port=5
  Camber : Constant  Value=0
  Constant : Constant  Value=Pacn
  Degrees to Radians : simulink_extras/Transformations/Degrees to Radians
  Degrees to Radians1 : simulink_extras/Transformations/Degrees to Radians
  Demux : Demux  Outputs=3
  Gain : Gain  Gain=-1
  Pacejka 96 : MATLAB Function  TreatAsAtomicUnit=on
  Terminator : Terminator
  Terminator1 : Terminator
  raggio ruota scarica [m] : Constant  Value=Rrear
  Fy : Outport  VectorParamsAs1DForOutWhenUnconnected=off
  Fx : Outport  Port=2  VectorParamsAs1DForOutWhenUnconnected=off
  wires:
  Demux/2 -> Gain/1  "Fy"
  Demux/1 -> Fx/1  "Fx"
  raggio ruota scarica [m]/1 -> Pacejka 96/8(R0)
  Degrees to Radians/1 -> Pacejka 96/2(gamma)
  Vcx/1 -> Pacejka 96/7(Vcx)
  Degrees to Radians1/1 -> Pacejka 96/4(alfa)
  Constant/1 -> Pacejka 96/1(Pac)
  Pacejka 96/1(F_pac) -> Demux/1
  Camber/1 -> Degrees to Radians/1
  s/1 -> Pacejka 96/3(slip)
  mu_strada/1 -> Pacejka 96/6(mu)
  alfa/1 -> Degrees to Radians1/1
  Fz/1 -> Pacejka 96/5(Fz)
  Pacejka 96/2(C_F) -> Terminator1/1
  Demux/3 -> Terminator/1  "Mz"
  Gain/1 -> Fy/1

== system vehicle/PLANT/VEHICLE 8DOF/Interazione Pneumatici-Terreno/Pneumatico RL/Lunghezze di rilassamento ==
  vel_x_CR : Inport
  Fy : Inport  Port=2
  Fx : Inport  Port=3
  Integrator : Integrator
  Integrator1 : Integrator
  Lunghezza di rilassamento longitudinale : Constant  Value=Lril_L
  Lunghezza di rilassamento trasversale : Constant  Value=Lril_T
  Math Function : Math  Operator=reciprocal  SignedPower=on
  Math Function1 : Math  Operator=reciprocal  SignedPower=on
  Product{,1..3} (4 alike) : Product  InputSameDT=on  SaturateOnIntegerOverflow=on
  Sum1 : Sum  Inputs=-+  InputSameDT=on  SaturateOnIntegerOverflow=on
  Sum2 : Sum  Inputs=-+  InputSameDT=on  SaturateOnIntegerOverflow=on
  Fy_rit : Outport  VectorParamsAs1DForOutWhenUnconnected=off
  Fx_rit : Outport  Port=2  VectorParamsAs1DForOutWhenUnconnected=off
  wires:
  Lunghezza di rilassamento longitudinale/1 -> Math Function/1
  Fx/1 -> Sum1/2
  Product/1 -> Product1/2
  Sum1/1 -> Product1/1
  Product1/1 -> Integrator/1
  Integrator/1 -> Fx_rit/1, Sum1/1
  vel_x_CR/1 -> Product/2, Product2/2
  Lunghezza di rilassamento trasversale/1 -> Math Function1/1
  Math Function1/1 -> Product2/1
  Fy/1 -> Sum2/2
  Product2/1 -> Product3/2
  Sum2/1 -> Product3/1
  Product3/1 -> Integrator1/1
  Integrator1/1 -> Fy_rit/1, Sum2/1
  Math Function/1 -> Product/1

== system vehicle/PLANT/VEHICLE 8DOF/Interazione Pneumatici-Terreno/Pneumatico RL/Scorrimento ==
  vel_x_cr : Inport
  R : Inport  Port=2
  w : Inport  Port=3
  Mux9 : Mux  Inputs=2
  Product : Product  InputSameDT=on  SaturateOnIntegerOverflow=on
  Switch : Switch
  slip frenata : Fcn  Expr=(u[2]/(u[1]+(u[1]==0)*eps))-1
  slip trazione : Fcn  Expr=1-(u[1]/(u[2]+(u[2]==0)*eps))
  s : Outport  VectorParamsAs1DForOutWhenUnconnected=off
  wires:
  slip frenata/1 -> Switch/3
  Mux9/1 -> slip frenata/1, slip trazione/1
  vel_x_cr/1 -> Mux9/1
  Switch/1 -> s/1
  Product/1 -> Mux9/2
  w/1 -> Product/1
  R/1 -> Product/2
  slip trazione/1 -> Switch/2, Switch/1

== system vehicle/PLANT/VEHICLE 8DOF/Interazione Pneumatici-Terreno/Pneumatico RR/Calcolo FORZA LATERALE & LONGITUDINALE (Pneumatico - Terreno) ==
  Vcx : Inport
  mu_strada : Inport  Port=2
  s : Inport  Port=3
  Fz : Inport  Port=4
  alfa : Inport  Port=5
  Camber : Constant  Value=0
  Constant : Constant  Value=Pacn
  Degrees to Radians : simulink_extras/Transformations/Degrees to Radians
  Degrees to Radians1 : simulink_extras/Transformations/Degrees to Radians
  Demux : Demux  Outputs=3
  Gain : Gain  Gain=-1
  Pacejka 96 : MATLAB Function  TreatAsAtomicUnit=on
  Terminator : Terminator
  Terminator1 : Terminator
  raggio ruota scarica [m] : Constant  Value=Rrear
  Fy : Outport  VectorParamsAs1DForOutWhenUnconnected=off
  Fx : Outport  Port=2  VectorParamsAs1DForOutWhenUnconnected=off
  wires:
  Demux/2 -> Gain/1  "Fy"
  Demux/1 -> Fx/1  "Fx"
  raggio ruota scarica [m]/1 -> Pacejka 96/8(R0)
  Degrees to Radians/1 -> Pacejka 96/2(gamma)
  Vcx/1 -> Pacejka 96/7(Vcx)
  Degrees to Radians1/1 -> Pacejka 96/4(alfa)
  Constant/1 -> Pacejka 96/1(Pac)
  Pacejka 96/1(F_pac) -> Demux/1
  Camber/1 -> Degrees to Radians/1
  s/1 -> Pacejka 96/3(slip)
  mu_strada/1 -> Pacejka 96/6(mu)
  alfa/1 -> Degrees to Radians1/1
  Fz/1 -> Pacejka 96/5(Fz)
  Pacejka 96/2(C_F) -> Terminator1/1
  Demux/3 -> Terminator/1  "Mz"
  Gain/1 -> Fy/1

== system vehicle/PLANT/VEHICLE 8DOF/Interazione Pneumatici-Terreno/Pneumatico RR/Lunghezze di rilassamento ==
  vel_x_CR : Inport
  Fy : Inport  Port=2
  Fx : Inport  Port=3
  Integrator : Integrator
  Integrator1 : Integrator
  Lunghezza di rilassamento longitudinale : Constant  Value=Lril_L
  Lunghezza di rilassamento trasversale : Constant  Value=Lril_T
  Math Function : Math  Operator=reciprocal  SignedPower=on
  Math Function1 : Math  Operator=reciprocal  SignedPower=on
  Product{,1..3} (4 alike) : Product  InputSameDT=on  SaturateOnIntegerOverflow=on
  Sum1 : Sum  Inputs=-+  InputSameDT=on  SaturateOnIntegerOverflow=on
  Sum2 : Sum  Inputs=-+  InputSameDT=on  SaturateOnIntegerOverflow=on
  Fy_rit : Outport  VectorParamsAs1DForOutWhenUnconnected=off
  Fx_rit : Outport  Port=2  VectorParamsAs1DForOutWhenUnconnected=off
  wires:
  Lunghezza di rilassamento longitudinale/1 -> Math Function/1
  Fx/1 -> Sum1/2
  Product/1 -> Product1/2
  Sum1/1 -> Product1/1
  Product1/1 -> Integrator/1
  Integrator/1 -> Fx_rit/1, Sum1/1
  vel_x_CR/1 -> Product/2, Product2/2
  Lunghezza di rilassamento trasversale/1 -> Math Function1/1
  Math Function1/1 -> Product2/1
  Fy/1 -> Sum2/2
  Product2/1 -> Product3/2
  Sum2/1 -> Product3/1
  Product3/1 -> Integrator1/1
  Integrator1/1 -> Fy_rit/1, Sum2/1
  Math Function/1 -> Product/1

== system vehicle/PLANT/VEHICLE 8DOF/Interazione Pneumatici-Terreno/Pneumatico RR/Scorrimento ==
  vel_x_cr : Inport
  R : Inport  Port=2
  w : Inport  Port=3
  Mux9 : Mux  Inputs=2
  Product : Product  InputSameDT=on  SaturateOnIntegerOverflow=on
  Switch : Switch
  slip frenata : Fcn  Expr=(u[2]/(u[1]+(u[1]==0)*eps))-1
  slip trazione : Fcn  Expr=1-(u[1]/(u[2]+(u[2]==0)*eps))
  s : Outport  VectorParamsAs1DForOutWhenUnconnected=off
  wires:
  slip frenata/1 -> Switch/3
  slip trazione/1 -> Switch/2, Switch/1
  Mux9/1 -> slip frenata/1, slip trazione/1
  vel_x_cr/1 -> Mux9/1
  Switch/1 -> s/1
  Product/1 -> Mux9/2
  w/1 -> Product/1
  R/1 -> Product/2

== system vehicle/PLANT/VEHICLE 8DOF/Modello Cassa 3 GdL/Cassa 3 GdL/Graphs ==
  vel : Inport
  beta : Inport  Port=2
  psi_p : Inport  Port=3
  a_y : Inport  Port=4
  teta : Inport  Port=5
  Gain1 : Gain  Gain=3.6
  Gain2 : Gain  Gain=1/g
  Integrator : Integrator
  Psi [°] 1 : Scope
  "Psi_p [°/s] " : Scope
  Radians to Degrees : simulink_extras/Transformations/Radians to Degrees
  Radians to Degrees1 : simulink_extras/Transformations/Radians to Degrees
  Radians to Degrees2 : simulink_extras/Transformations/Radians to Degrees
  "Vel [km/h] " : Scope
  "ay " : Scope
  beta [°] : Scope
  "teta [°] " : Scope
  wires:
  Radians to Degrees1/1 -> Integrator/1, "Psi_p [°/s] "/1
  Gain1/1 -> "Vel [km/h] "/1
  Radians to Degrees/1 -> beta [°]/1
  Radians to Degrees2/1 -> "teta [°] "/1
  vel/1 -> Gain1/1
  beta/1 -> Radians to Degrees/1
  psi_p/1 -> Radians to Degrees1/1
  a_y/1 -> Gain2/1
  teta/1 -> Radians to Degrees2/1
  Gain2/1 -> "ay "/1
  Integrator/1 -> Psi [°] 1/1

== matlab function vehicle/PLANT/VEHICLE 8DOF/Interazione 
Pneumatici-Terreno/Pneumatico FL/Calcolo FORZA LATERALE & LONGITUDINALE
(Pneumatico - Terreno)/Pacejka 96 ==
function [F_pac,C_F] = fcn(Pac,gamma,slip,alfa,Fz,mu,Vcx,R0)
% function x il calcolo delle forze Fx, Fy e Mz

% Pac   -> struttura con coeff. Pacejka 96
% slip     -> scorrimento
% alfa  -> deriva [rad]
% gamma -> camber [rad]
% Vcx,y componenti della velocita' del centro di contatto C della ruota

% Ricostruzione struttura: coefficienti modello 
Pa_FZ0_ = Pac(1);
Pa_LFZ0 = Pac(2);
Pa_LmuV = Pac(3);
Pa_LKXK = Pac(4);
Pa_LKYA = Pac(5);
Pa_LCX_ = Pac(6);
Pa_LCY_ = Pac(7);
Pa_LEX_ = Pac(8);
Pa_LEY_ = Pac(9);
Pa_LHX_ = Pac(10);
Pa_LHY_ = Pac(11);
Pa_LVX_ = Pac(12);
Pa_LVY_ = Pac(13);
Pa_LKYG = Pac(14);
Pa_LKZG = Pac(15);
Pa_LT__ = Pac(16);
Pa_MR__ = Pac(17);
Pa_LXA_ = Pac(18);
Pa_LYK_ = Pac(19);
Pa_LVYK = Pac(20);
Pa_LS__ = Pac(21);
Pa_LCZ_ = Pac(22);
Pa_LMX_ = Pac(23);
Pa_LMY_ = Pac(24);
Pa_PCX1 = Pac(25);
Pa_PDX1 = Pac(26);
Pa_PDX2 = Pac(27);
Pa_PEX1 = Pac(28);
Pa_PEX2 = Pac(29);
Pa_PEX3 = Pac(30);
Pa_PEX4 = Pac(31);
Pa_PKX1 = Pac(32);
Pa_PKX2 = Pac(33);
Pa_PKX3 = Pac(34);
Pa_PHX1 = Pac(35);
Pa_PHX2 = Pac(36);
Pa_PVX1 = Pac(37);
Pa_PVX2 = Pac(38);
Pa_RBX1 = Pac(39);
Pa_RBX2 = Pac(40);
Pa_RCX1 = Pac(41);
Pa_RHX1 = Pac(42);
Pa_RTX1 = Pac(43);
Pa_RTX2 = Pac(44);
Pa_RTX3 = Pac(45);
Pa_QSX1 = Pac(46);
Pa_QSX2 = Pac(47);
Pa_QSX3 = Pac(48);
Pa_PCY1 = Pac(49);
Pa_PDY1 = Pac(50);
Pa_PDY2 = Pac(51);
Pa_PDY3 = Pac(52);
Pa_PEY1 = Pac(53);
Pa_PEY2 = Pac(54);
Pa_PEY3 = Pac(55);
Pa_PEY4 = Pac(56);
Pa_PKY1 = Pac(57);
Pa_PKY2 = Pac(58);
Pa_PKY3 = Pac(59);
Pa_PHY1 = Pac(60);
Pa_PHY2 = Pac(61);
Pa_PHY3 = Pac(62);
Pa_PVY1 = Pac(63);
Pa_PVY2 = Pac(64);
Pa_PVY3 = Pac(65);
Pa_PVY4 = Pac(66);
Pa_RBY1 = Pac(67);
Pa_RBY2 = Pac(68);
Pa_RBY3 = Pac(69);
Pa_RCY1 = Pac(70);
Pa_RHY1 = Pac(71);
Pa_RVY1 = Pac(72);
Pa_RVY2 = Pac(73);
Pa_RVY3 = Pac(74);
Pa_RVY4 = Pac(75);
Pa_RVY5 = Pac(76);
Pa_RVY6 = Pac(77);
Pa_PTY1 = Pac(78);
Pa_PTY2 = Pac(79);
Pa_QSY1 = Pac(80);
Pa_QSY2 = Pac(81);
Pa_QBZ1 = Pac(82);
Pa_QBZ2 = Pac(83);
Pa_QBZ3 = Pac(84);
Pa_QBZ4 = Pac(85);
Pa_QBZ5 = Pac(86);
Pa_QBZ6 = Pac(87);
Pa_QBZ9 = Pac(88);
Pa_QBZZ = Pac(89);
Pa_QCZ1 = Pac(90);
Pa_QDZ1 = Pac(91);
Pa_QDZ2 = Pac(92);
Pa_QDZ3 = Pac(93);
Pa_QDZ4 = Pac(94);
Pa_QDZ6 = Pac(95);
Pa_QDZ7 = Pac(96);
Pa_QDZ8 = Pac(97);
Pa_QDZ9 = Pac(98);
Pa_QEZ1 = Pac(99);
Pa_QEZ2 = Pac(100);
Pa_QEZ3 = Pac(101);
Pa_QEZ4 = Pac(102);
Pa_QEZ5 = Pac(103);
Pa_QHZ1 = Pac(104);
Pa_QHZ2 = Pac(105);
Pa_QHZ3 = Pac(106);
Pa_QHZ4 = Pac(107);
Pa_SSZ1 = Pac(108);
Pa_SSZ2 = Pac(109);
Pa_SSZ3 = Pac(110);
Pa_SSZ4 = Pac(111);
Pa_QTZ1 = Pac(112);

% Costanti
epsi = 0.01;
eps_V = 0.1;
csi_0=1;
csi_4=1;
Amu = 10;
Pa_LmuX = mu;
Pa_LmuY = mu;

%-------------------------------- Fx pure slip ---------------------------
Cx = Pa_PCX1*Pa_LCX_;
dfz = (Fz-Pa_LFZ0*Pa_FZ0_)/(Pa_LFZ0*Pa_FZ0_);
mux = Pa_LmuX * (Pa_PDX1 + Pa_PDX2 * dfz);
Dx = mux*Fz; %*csi_1, con csi_1=1
%Shx = (Pa_PHX1+Pa_PHX2*dfz)*Pa_LHX_;
Shx = 0;
Kx = slip + Shx;
Ex = (Pa_PEX1+Pa_PEX2*dfz+Pa_PEX3*dfz^2)*(1-Pa_PEX4*sign(Kx))*Pa_LEX_;
if Ex>1 Et=1; end
Kxk = Fz*(Pa_PKX1+Pa_PKX2*dfz)*exp(Pa_PKX3*dfz)*Pa_LKXK;
Bx = Kxk/(Cx*Dx+epsi);
lam_mux  = Pa_LmuX*Amu/(1+(Amu-1)*Pa_LmuX);
SVx = Fz*(Pa_PVX1+Pa_PVX2*dfz)*(abs(Vcx)/(abs(Vcx)+eps_V))*Pa_LVX_*lam_mux; %*csi_1, con csi_1=1

% logitudinal slip stiffness (pendenza curva Fx nell'origine)
C_Fk = Bx*Cx*Dx;

% Forza longitudinale
Fx0 = Dx*sin(Cx*atan(Bx*Kx-Ex*(Bx*Kx-atan(Bx*Kx)))) + SVx;

%---------------------------- Fy pure side slip --------------------------
seg=sign(Vcx);
if seg==0 seg=1; end
alfa_star = tan(alfa)*seg;
gam_star = sin(gamma);
Shy = (Pa_PHY1+Pa_PHY2*dfz)*Pa_LHY_+Pa_PHY3*gam_star*Pa_LKYG*csi_0+csi_4-1;
alfa_y = alfa_star + Shy;
Cy = Pa_PCY1*Pa_LCY_;
muy = Pa_LmuY*(Pa_PDY1+Pa_PDY2*dfz)*(1-Pa_PDY3*gam_star^2);
Dy = muy*Fz; %*csi_2, con csi_2=1
Ey = (Pa_PEY1+Pa_PEY2*dfz)*(1-(Pa_PEY3+Pa_PEY4*gam_star)*sign(alfa_y))*Pa_LEY_;
if Ey>1 Ey=1; end
Kya0 = Pa_PKY1*Pa_LFZ0*Pa_FZ0_*sin(2*atan(Fz/(Pa_PKY2*Pa_LFZ0*Pa_FZ0_)))*Pa_LKYA;
Kya = Kya0*(1-Pa_PKY3*gam_star^2); %*csi_3, con csi_3=1
By = Kya/(Cy*Dy+epsi);
lam_muy = Pa_LmuY*Amu/(1+(Amu-1)*Pa_LmuY);
SVy = Fz*((Pa_PVY1+Pa_PVY2*dfz)*Pa_LVY_+(Pa_PVY3+Pa_PVY4*dfz)*gam_star*Pa_LKYG )*lam_muy; %*csi_2, con csi_2=1
Kyg0 = (Pa_PHY3*Kya0+Fz*(Pa_PVY3+Pa_PVY4*dfz))*Pa_LKYG;

% cornering stiffness (pendenza curva Fy nell'origine)
C_Fa = By*Cy*Dy;

% Forza laterale
Fy0 = Dy*sin(Cy*atan(By*alfa_y-Ey*(By*alfa_y-atan(By*alfa_y)))) + SVy;

% --------------------- Fx combined slip ------------------------------
Shxa = Pa_RHX1;
%Exa = Pa_REX1+Pa_REX2*dfz; NON esiste Pa.REX1 ne' Pa.REX2
Exa = 0;
Cxa = Pa_RCX1;
Bxa = Pa_RBX1*cos(atan(Pa_RBX2*slip))*Pa_LXA_;
alfaS = alfa_star+Shxa;
Gxa0 = cos(Cxa*atan(Bxa*Shxa-Exa*(Bxa*Shxa-atan(Bxa*Shxa))));
Gxa = cos(Cxa*atan(Bxa*alfaS-Exa*(Bxa*alfaS-atan(Bxa*alfaS))))/Gxa0;
Fx = Fx0*Gxa;

% ---------------------- Fy combined slip ------------------------------
Dvyk = muy*Fz*(Pa_RVY1+Pa_RVY2*dfz+Pa_RVY3*gam_star)*cos(atan(Pa_RVY4*alfa_star));%*csi_2, con csi_2=1
Svyk = Dvyk*sin(Pa_RVY5*atan(Pa_RVY6*slip));
Shyk = Pa_RHY1; %+Pa.RHY2*dfz; NON esiste Pa.RHY2
Cyk = Pa_RCY1;
Byk = Pa_RBY1*cos(atan(Pa_RBY2*(alfa_star-Pa_RBY3)))*Pa_LYK_;
%Eyk = Pa_REY1+Pa_REY2*dfz; NON esiste Pa.REY1 ne' Pa.REY2
Eyk = 0;
ks = slip+Shyk;
Gyk0 = cos(Cyk*atan(Byk*Shyk-Eyk*(Byk*Shyk-atan(Byk*Shyk))));
Gyk = cos(Cyk*atan(Byk*ks-Eyk*(Byk*ks-atan(Byk*ks))))/Gyk0;
Fy = Fy0*Gyk+Svyk;

% --------------------- Mz pure side slip  ---------------------------
Shf = Shy+SVy/Kya;
alfa_r = alfa_star+Shf;
Br = (Pa_QBZ9/Pa_LmuY+Pa_QBZZ*By*Cy); %*csi_6, con csi_6=1
%%% Pa_QBZZ e' in realta' QBZ10 scritto cosi' x ragioni di spazio
Cr = 1; %*csi_7, con csi_7=1
Dr = Fz*R0*((Pa_QDZ6+Pa_QDZ7*dfz)+(Pa_QDZ8+Pa_QDZ9*dfz)*gam_star)*cos(alfa)*Pa_LmuY*seg; %+csi_8-1, con csi_8=1
Mzr0 = Dr*cos(Cr*atan(Br*alfa_r));
Sht = Pa_QHZ1+Pa_QHZ2*dfz+(Pa_QHZ3+Pa_QHZ4*dfz)*gam_star;
alfa_t = alfa_star+Sht;
Bt = (Pa_QBZ1+Pa_QBZ2*dfz+Pa_QBZ3*dfz^2)*(1+Pa_QBZ5*abs(gam_star)+Pa_QBZ6*gam_star^2)*Pa_LKYA/Pa_LmuY;
if Bt<0 Bt=0; end
Ct = Pa_QCZ1;
Dt0 = Fz*R0/(Pa_LFZ0*Pa_FZ0_)*(Pa_QDZ1+Pa_QDZ2*dfz)*seg;
Dt = Dt0*(1+Pa_QDZ3*abs(gam_star)+Pa_QDZ4*gam_star^2); %*csi_5, con csi_5=1
Et = (Pa_QEZ1+Pa_QEZ2*dfz+Pa_QEZ3*dfz^2)*(1+(Pa_QEZ4+Pa_QEZ5*gam_star)*2/pi*atan(Bt*Ct*alfa_t));
if Et>1 Et=1; end
t0 = Dt*cos(Ct*atan(Bt*alfa_t - Et*(Bt*alfa_t-atan(Bt*alfa_t))))*cos(alfa);
Mz0 = -t0*Fy;
Kza0 = Dt0*Kya0;
%Kzg0 = Fz*R0*(Pa_QDZ8+Pa_QDZ9*dfz)-Dt0*Kyg0;

% momento autoallineamento (aligning torque)
Mz = Mz0 + Mzr0;

% ------------------------ Mz Combined -----------------------------
eps_k = 0; % ???????
lambda_s = Pa_LS__ ;
Fz0p = Pa_LFZ0*Pa_FZ0_;
K_yap = Kya + eps_k;
alfa_req = sqrt(alfa_r^2+(Kxk/K_yap)^2*slip^2)*sign(alfa_r);
alfa_teq = sqrt(alfa_t^2+(Kxk/K_yap)^2*slip^2)*sign(alfa_t);
s = R0*(Pa_SSZ1 + Pa_SSZ2*(Fy/Fz0p) + (Pa_SSZ3+Pa_SSZ4*dfz)*gam_star)*lambda_s;
Mzr = Dr*cos(Cr*atan(Br*alfa_req));
Fyp = Fy-Svyk; 
t = Dt*cos(Ct*atan(Bt*alfa_teq - Et*(Bt*alfa_teq-atan(Bt*alfa_teq))))*cos(alfa);
Mzp = -t*Fyp;
% momento autoallineamento (aligning torque)
Mz = Mzp + Mzr + s*Fx;
%%%%%%%%%%%%%%%%%%%%%%%

% Controllo che forza verticale Fz sia positiva
if Fz <= 0
    Fx = 0;
    Fy = 0;
    Mz = 0;
end

% Output
F_pac = [Fx; Fy; Mz];
C_F = [C_Fk; C_Fa];
